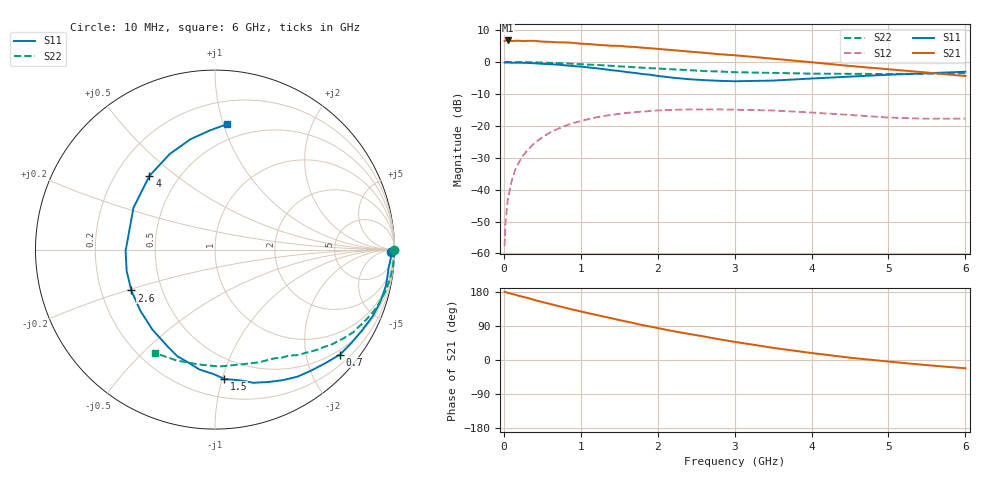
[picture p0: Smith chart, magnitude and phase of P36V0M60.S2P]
! SIEMENS Small Signal Semiconductors
! BFP181
! Si NPN RF Bipolar Junction Transistor in SOT143
! VCE = 6 V  IC = 0.6 mA
! Common Emitter S-Parameters:  March  1996
# GHz  S  MA  R  50
!  f  S11  S21  S12  S22
! GHz  MAG  ANG  MAG  ANG  MAG  ANG  MAG  ANG
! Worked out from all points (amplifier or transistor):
!   36 points, 10 MHz to 6 GHz, reference 50 ohm
!   highest |S21| = 6.7 dB at 50 MHz (marker M1)
!   |S21| within 3 dB of that: start of sweep to 2.177 GHz
!   unconditionally stable (mu >= 1): 3.711 GHz to end of sweep
!   at 250 MHz: K = 0.08, MSG = 17.9 dB, |S12| = -29.4 dB
!   at 1.4 GHz: K = 0.43, MSG = 10.8 dB, |S12| = -16.6 dB
!   at 6 GHz: K = 1.39, MAG = 3.0 dB, |S12| = -17.8 dB
!   S11 on the Smith chart (normalised r, x): 10 MHz: 69, -38; 700 MHz: 0.40, -2.70; 1.5 GHz: 0.34, -1.02; 2.6 GHz: 0.33, -0.21; 4 GHz: 0.34, +0.40; 6 GHz: 0.37, +1.03
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0.01  0.978 -0.7  2.139 179.7  0.0013 87.4  0.9993 -0.2
0.02  0.9819 -1.2  2.155 179.5  0.0029 86.3  0.9982 -0.5
0.05  0.9807 -2.8  2.171 177.3  0.0068 91.9  0.9973 -1.4
0.1  0.973 -5.8  2.123 174.7  0.0135 85.4  0.9982 -2.8
0.15  0.9723 -8.8  2.147 172.0  0.0207 83.4  0.996 -4.2
0.25  0.9698 -14.3  2.119 166.6  0.034 80.1  0.9928 -6.9
0.3  0.9661 -17.6  2.137 164.3  0.0406 78.0  0.9903 -8.3
0.4  0.9534 -23.0  2.139 158.2  0.0537 74.1  0.9847 -11.0
0.7  0.9097 -40.0  2.028 142.8  0.0892 62.3  0.9586 -18.9
0.9  0.8619 -51.3  1.991 132.7  0.11 54.5  0.934 -23.8
1.1  0.82 -62.5  1.914 123.4  0.1272 47.8  0.9081 -28.4
1.5  0.7226 -85.8  1.788 105.4  0.1539 35.2  0.8525 -36.7
1.8  0.6469 -103.2  1.673 92.2  0.1666 27.3  0.8123 -42.1
1.9  0.63 -109.5  1.642 88.5  0.1703 24.2  0.8 -44.0
2.2  0.5659 -128.1  1.529 76.1  0.1774 17.2  0.7653 -48.8
2.6  0.5188 -154.0  1.393 62.1  0.1799 9.2  0.72 -55.0
3  0.4981 -179.1  1.274 47.9  0.1786 1.4  0.6909 -61.2
3.5  0.5107 152.8  1.124 32.1  0.1737 -5.7  0.6735 -68.8
4  0.5497 131.6  0.989 18.4  0.1612 -11.2  0.6552 -77.9
4.5  0.5894 115.3  0.865 6.1  0.1479 -14.7  0.6516 -88.0
5.5  0.6645 92.5  0.682 -13.6  0.1289 -11.0  0.6538 -109.0
6  0.7028 84.4  0.602 -21.9  0.1292 -7.8  0.6653 -119.9
